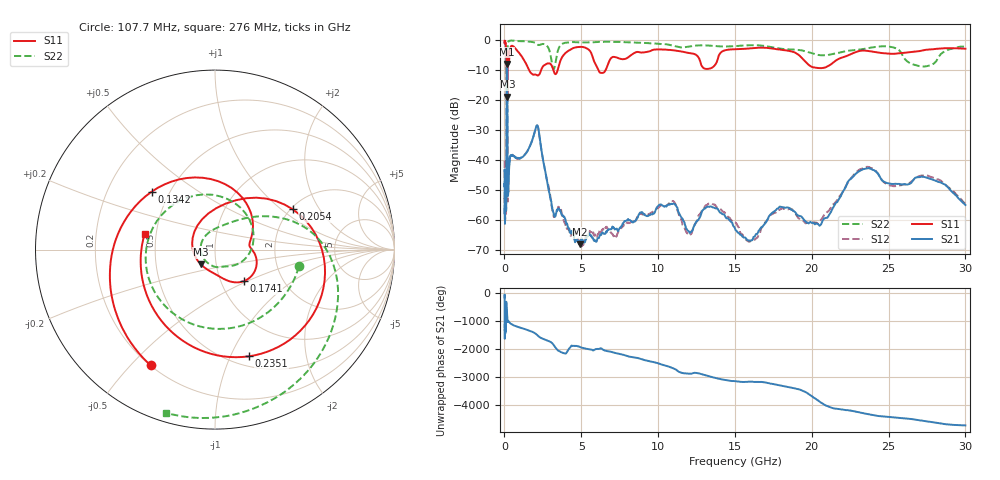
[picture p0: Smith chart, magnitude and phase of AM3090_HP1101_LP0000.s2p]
! Date/Time: Thu, Feb 28, 2019 2:07 PM
! Network Analyzer: Agilent Technologies E8364B Rev: A.07.50.67
! Sweep from 0.010 to 30.000 GHz, 1601 Points, Sweep Type: LOG
! Power Supply: 5.023 V, 0.002 A
# Hz S DB R 50
!freq MagS11 AngS11 MagS21 AngS21 MagS12 AngS12 MagS22 AngS22
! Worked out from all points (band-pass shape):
!   1601 points, 10 MHz to 30 GHz, reference 50 ohm
!   highest |S21| = -7.99 dB at 162.4 MHz (marker M1); lowest = -68.0 dB at 4.927 GHz (marker M2)
!   |S21| within 3 dB of the highest: 147.9 MHz to 180.4 MHz (32.46 MHz wide, 19.8 % of centre)
!   lowest |S11| = -18.9 dB at 186.8 MHz (marker M3), VSWR 1.26, Z = 42.1 - j7.02 ohm
!   |S11| at or under -10 dB: 1.604 GHz to 2.383 GHz (779.2 MHz wide, 39.1 % of centre); 3.188 GHz to 3.462 GHz (274.3 MHz wide, 8.25 % of centre); 6.112 GHz to 6.585 GHz (473.2 MHz wide, 7.45 % of centre)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
!   |S22| runs from -22.0 to -0.1 dB; largest |S21 - S12| = 0.016
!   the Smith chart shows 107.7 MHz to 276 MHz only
!   S11 on the Smith chart (normalised r, x): 107.7 MHz: 0.20, -0.57; 134.2 MHz: 0.40, +0.33; 174.1 MHz: 1.28, -0.48; 205.4 MHz: 2.05, +1.21; 235.1 MHz: 0.60, -1.17; 276 MHz: 0.43, +0.09
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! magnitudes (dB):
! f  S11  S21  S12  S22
! 10 MHz  -0.3  -43.4  -40.2  -0.5
! 38.04 MHz  -0.3  -59.5  -57.5  -1.1
! 47.89 MHz  -0.5  -51.7  -47.8  -1.3
! 107.7 MHz  -2.6  -55.8  -56.0  -6.4
! 134.2 MHz  -6.4  -26.8  -26.7  -9.3
! 144.7 MHz  -10.5  -13.3  -13.3  -13.4
! 162.4 MHz  -12.9  -8.0  -7.9  -20.2
! 174.1 MHz  -12.5  -9.1  -9.0  -21.2
! 186.8 MHz  -18.9  -15.9  -15.8  -12.0
! 205.4 MHz  -6.2  -46.8  -45.4  -2.7
! 235.1 MHz  -4.1  -50.4  -52.5  -0.8
! 276 MHz  -7.9  -46.4  -45.9  -0.4
! 550.5 MHz  -2.1  -38.5  -38.4  -0.2
! 2.084 GHz  -11.6  -28.6  -28.6  -1.2
! 3.172 GHz  -9.7  -57.2  -57.9  -9.5
! 4.927 GHz  -2.3  -68.0  -68.3  -0.8
! 7.926 GHz  -6.2  -60.2  -61.1  -0.7
! 13.54 GHz  -9.1  -55.7  -54.6  -1.9
! 16.05 GHz  -2.7  -66.7  -66.6  -1.7
! 20.51 GHz  -9.4  -61.8  -60.3  -5.0
! 23.48 GHz  -3.5  -42.9  -42.4  -2.9
! 30 GHz  -2.9  -54.9  -54.5  -2.2
